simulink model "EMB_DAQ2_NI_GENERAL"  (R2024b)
settings: Solver=ode4  StartTime=0.0  StopTime=S  FixedStep=T  RelTol=1e-3  EnableMultiTasking=on
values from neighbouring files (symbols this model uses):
  T = 0.001    [EMB_DAQ2_NI_GENERAL_script.m]
undefined symbols (not defined in the file or in its folder): National_Instruments, PCIe
libraries: sldrtlib x5

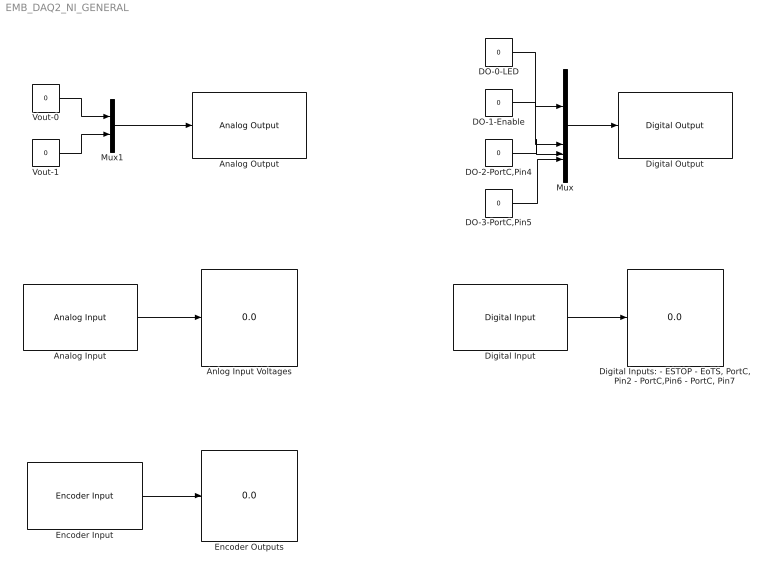
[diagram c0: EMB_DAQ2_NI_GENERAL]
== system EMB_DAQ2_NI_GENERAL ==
  Analog Input : sldrtlib/Analog Input  SampleTime=T  MaxMissedTicks=10  ShowMissedTicks=off  YieldWhenWaiting=off  DrvName=National_Instruments/PCIe-6321  DrvAddress=4294967295  DrvOptions=[0 15 0 2 2 2 2]  Channels=[1,2,3,4]  RangeMode=1  VoltRange=1  DataType=1
  Analog Output : sldrtlib/Analog Output  SampleTime=T  MaxMissedTicks=10  ShowMissedTicks=off  YieldWhenWaiting=off  DrvName=National_Instruments/PCIe-6321  DrvAddress=4294967295  DrvOptions=[0 15 0 2 2 2 2]  Channels=[1,2]  RangeMode=1  VoltRange=1  InitialValue=0  FinalValue=0
  Anlog Input Voltages : Display
  DO-0-LED : Constant  Value=0  OutDataTypeStr=double
  DO-1-Enable : Constant  Value=0  OutDataTypeStr=double
  DO-2-PortC,Pin4 : Constant  Value=0  OutDataTypeStr=double
  DO-3-PortC,Pin5 : Constant  Value=0  OutDataTypeStr=double
  Digital Input : sldrtlib/Digital Input  SampleTime=T  MaxMissedTicks=10  ShowMissedTicks=off  YieldWhenWaiting=off  DrvName=National_Instruments/PCIe-6321  DrvAddress=4294967295  DrvOptions=[0 15 0 2 2 2 2]  Channels=[5,6,7,8]  BitMode=1  DataType=1
  "Digital Inputs: - ESTOP - EoTS, PortC, Pin2 - PortC,Pin6 - PortC, Pin7" : Display
  Digital Output : sldrtlib/Digital Output  SampleTime=T  MaxMissedTicks=10  ShowMissedTicks=off  YieldWhenWaiting=off  DrvName=National_Instruments/PCIe-6321  DrvAddress=4294967295  DrvOptions=[0 15 0 2 2 2 2]  Channels=[1,2,3,4]  BitMode=1  InitialValue=0  FinalValue=0
  Encoder Input : sldrtlib/Encoder Input  SampleTime=T  MaxMissedTicks=10  ShowMissedTicks=off  YieldWhenWaiting=off  DrvName=National_Instruments/PCIe-6321  DrvAddress=4294967295  DrvOptions=[0 15 0 2 2 2 2]  Channels=[1,2,3,4]  QuadMode=3  IndexPulse=1  InputFilter=Inf  DataType=1
  Encoder Outputs : Display
  Mux : Mux
  Mux1 : Mux  Inputs=2
  Vout-0 : Constant  Value=0  OutDataTypeStr=double
  Vout-1 : Constant  Value=0  OutDataTypeStr=double
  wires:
  Encoder Input/1 -> Encoder Outputs/1
  DO-1-Enable/1 -> Mux/2
  DO-0-LED/1 -> Mux/1
  Mux/1 -> Digital Output/1
  Mux1/1 -> Analog Output/1
  Vout-0/1 -> Mux1/1
  Vout-1/1 -> Mux1/2
  DO-3-PortC,Pin5/1 -> Mux/4
  DO-2-PortC,Pin4/1 -> Mux/3
  Digital Input/1 -> "Digital Inputs: - ESTOP - EoTS, PortC, Pin2 - PortC,Pin6 - PortC, Pin7"/1
  Analog Input/1 -> Anlog Input Voltages/1
